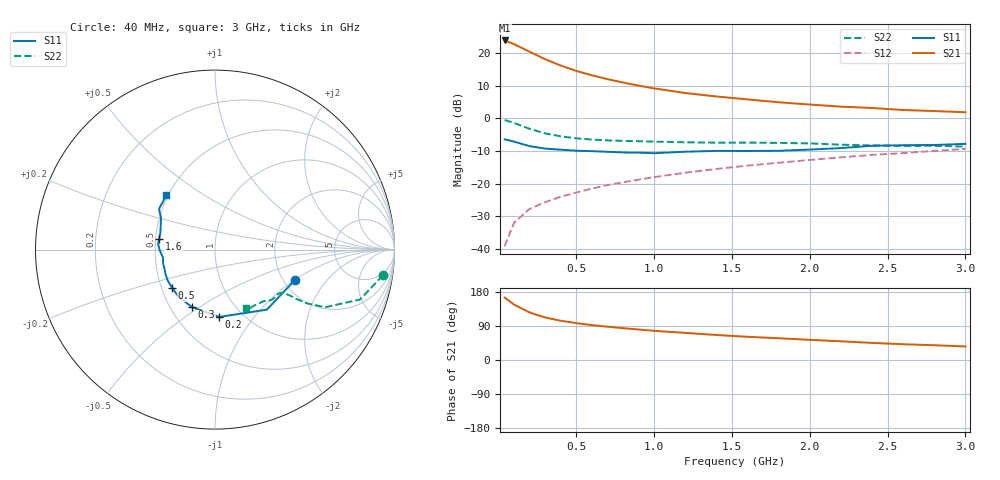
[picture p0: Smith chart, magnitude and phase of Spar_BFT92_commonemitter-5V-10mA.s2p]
! Filename:  BFT92C.S2P  Version:  2.0
! NXP part #: BFT92  Date: May 1990
! Bias condition: Vce=-5V, Ic=-10mA
#  MHz  S  MA  R  50
! Freq  S11  S21  S12  S22  !GUM [dB]
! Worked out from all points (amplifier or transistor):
!   21 points, 40 MHz to 3 GHz, reference 50 ohm
!   highest |S21| = 23.9 dB at 40 MHz (marker M1)
!   |S21| within 3 dB of that: start of sweep to 180.6 MHz
!   unconditionally stable (mu >= 1): 724.4 MHz to 2.282 GHz
!   at 300 MHz: K = 0.74, MSG = 21.9 dB, |S12| = -25.7 dB
!   at 1 GHz: K = 1.07, MAG = 12.0 dB, |S12| = -18.0 dB
!   at 3 GHz: K = 0.93, MSG = 5.6 dB, |S12| = -9.3 dB
!   S11 on the Smith chart (normalised r, x): 40 MHz: 2.32, -1.00; 200 MHz: 0.78, -0.69; 300 MHz: 0.64, -0.47; 500 MHz: 0.57, -0.27; 1.6 GHz: 0.52, +0.07; 3 GHz: 0.49, +0.35
40  0.478 -20.4  15.7 164.7  0.011 81.7  0.947 -8.7
100  0.442 -49.2  13.81 146.4  0.025 72.5  0.854 -19.0
200  0.376 -86.4  10.55 125.4  0.041 65.7  0.693 -27.6
300  0.345 -111.8  8.101 112.3  0.052 64.2  0.591 -30.4
400  0.332 -127.7  6.478 103.6  0.063 64.7  0.531 -31.2
500  0.32 -138.3  5.361 97.3  0.073 65.9  0.495 -31.5
600  0.315 -146.6  4.588 92.1  0.084 66.7  0.475 -31.8
700  0.308 -153.3  4.006 88.0  0.095 67.7  0.461 -32.0
800  0.301 -159.1  3.558 84.0  0.105 68.5  0.453 -32.1
900  0.299 -165.3  3.188 80.5  0.115 68.8  0.448 -32.5
1000  0.293 -171.1  2.889 77.0  0.126 69.0  0.441 -33.1
1200  0.309 -179.7  2.456 71.6  0.147 69.3  0.431 -34.7
1400  0.318 174.6  2.173 66.0  0.168 69.3  0.425 -37.1
1600  0.317 168.9  1.959 61.2  0.189 68.8  0.426 -39.4
1800  0.319 162.5  1.77 57.4  0.209 68.8  0.422 -41.5
2000  0.333 155.1  1.634 53.2  0.231 68.0  0.414 -43.4
2200  0.351 149.1  1.516 49.4  0.253 67.6  0.396 -46.3
2400  0.381 144.7  1.446 45.1  0.276 66.6  0.386 -51.2
2600  0.388 142.7  1.347 41.6  0.294 65.8  0.38 -56.0
2800  0.392 138.3  1.298 39.0  0.318 65.4  0.381 -59.3
3000  0.407 132.0  1.245 35.7  0.341 64.4  0.37 -61.9
